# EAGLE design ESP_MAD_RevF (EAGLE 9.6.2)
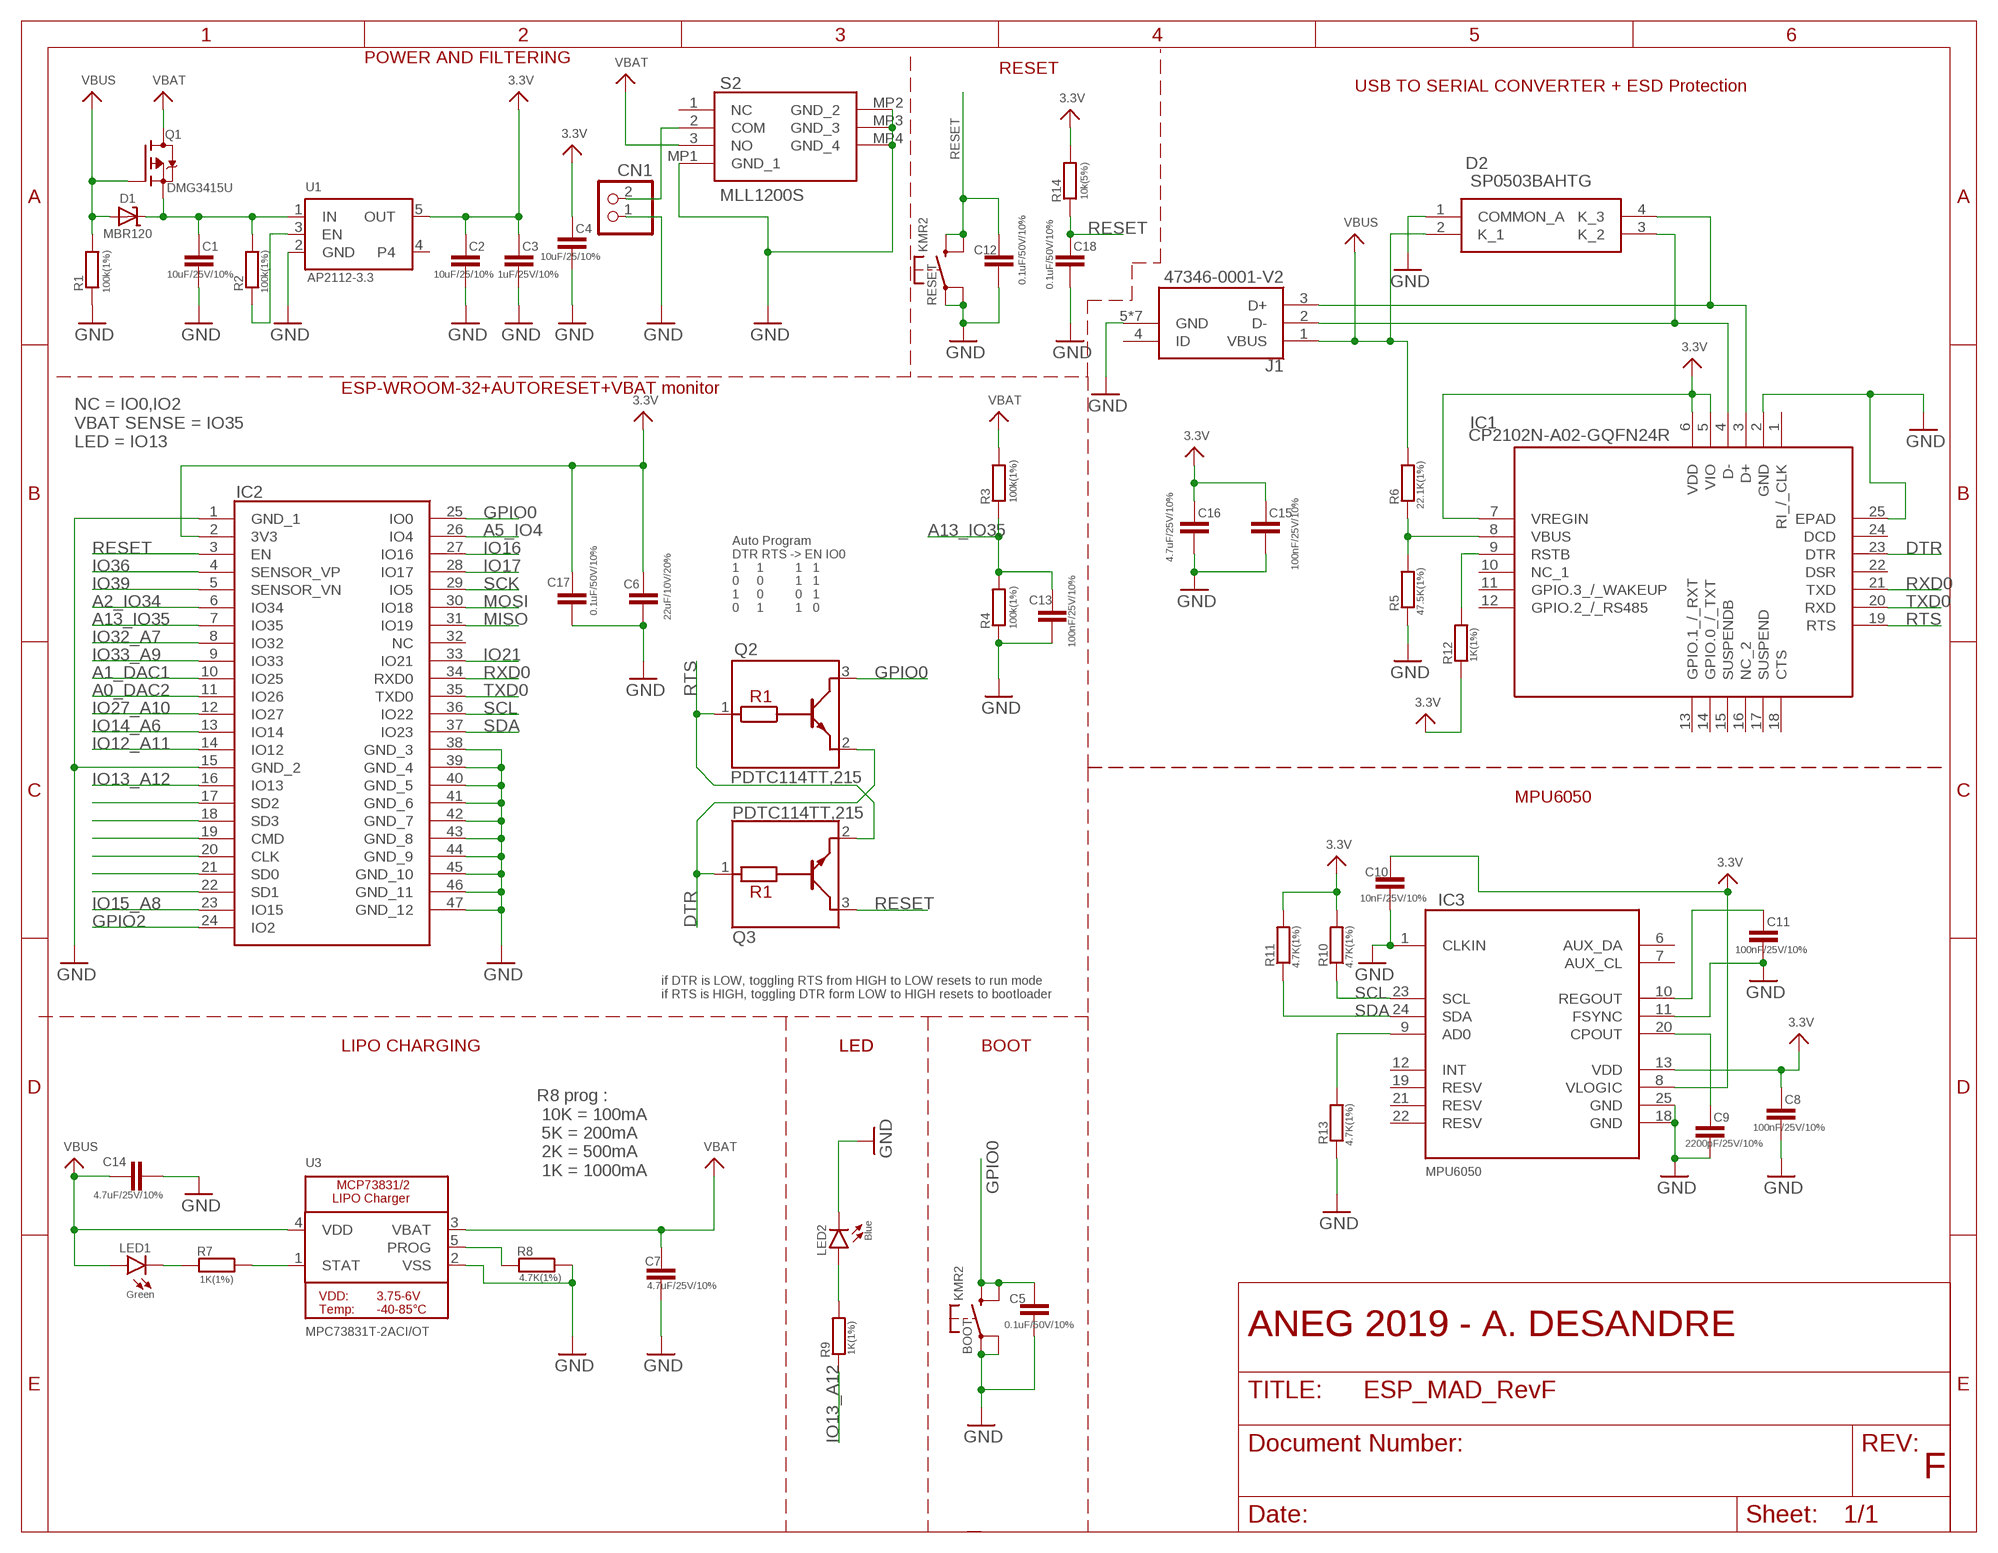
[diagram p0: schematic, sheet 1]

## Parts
BOOT  KMR2  MICROBUILDER_SWITCH_TACT_SMT4.6X2.8  [MICROBUILDER_BTN_KMR2_4.6X2.8]
C1  10uF/25V/10%  C-EUC0603  [C0603]
C2  10uF/25/10%  C-EUC0603  [C0603]
C3  1uF/25V/10%  C-EUC0603  [C0603]
C4  10uF/25/10%  C-EUC0603  [C0603]
C5  0.1uF/50V/10%  C-EUC0603  [C0603]
C6  22uF/10V/20%  C-EUC0603  [C0603]
C7  4.7uF/25V/10%  C-EUC0603  [C0603]
C8  100nF/25V/10%  C-EUC0603  [C0603]
C9  2200pF/25V/10%  C-EUC0603  [C0603]
C10  10nF/25V/10%  C-EUC0603  [C0603]
C11  100nF/25V/10%  C-EUC0603  [C0603]
C12  0.1uF/50V/10%  C-EUC0603  [C0603]
C13  100nF/25V/10%  C-EUC0603  [C0603]
C14  4.7uF/25V/10%  C-EUC0603  [C0603]
C15  100nF/25V/10%  C-EUC0603  [C0603]
C16  4.7uF/25V/10%  C-EUC0603  [C0603]
C17  0.1uF/50V/10%  C-EUC0603  [C0603]
C18  0.1uF/50V/10%  C-EUC0603  [C0603]
CN1  JST_2PIN-SMT-RA  [JST-PH-2-SMT-RA]
D1  MBR120  MICROBUILDER_DIODE-SCHOTTKYSOD-123  [MICROBUILDER_SOD-123]
D2  SP0503BAHTG  [SP0503BAHTG]
IC1  CP2102N-A02-GQFN24R  [QFN50P400X400X80-25N]
IC2  ESP32-WROOM-32D_M113DH3200PS3Q  [ESP32WROOM32DM113DH3200PS3Q0]
IC3  MPU6050  [QFN50P400X400X95-25T265X275N]
J1  47346-0001-V2  [47346-0001-V2]
LED1  Green  LEDCHIP-LED0603  [CHIP-LED0603]
LED2  Blue  LEDCHIP-LED0603  [CHIP-LED0603]
Q1  DMG3415U  MICROBUILDER_MOSFET-P  [MICROBUILDER_SOT23-R]
Q2  PDTC114TT,215  [SOT95P230X110-3N]
Q3  PDTC114TT,215  [SOT95P230X110-3N]
R1  100k(1%)  R-EU_R0603  [R0603]
R2  100k(1%)  R-EU_R0603  [R0603]
R3  100k(1%)  R-EU_R0603  [R0603]
R4  100k(1%)  R-EU_R0603  [R0603]
R5  47.5K(1%)  R-EU_R0603  [R0603]
R6  22.1K(1%)  R-EU_R0603  [R0603]
R7  1K(1%)  R-EU_R0603  [R0603]
R8  4.7K(1%)  R-EU_R0603  [R0603]
R9  1K(1%)  R-EU_R0603  [R0603]
R10  4.7K(1%)  R-EU_R0603  [R0603]
R11  4.7K(1%)  R-EU_R0603  [R0603]
R12  1K(1%)  R-EU_R0603  [R0603]
R13  4.7K(1%)  R-EU_R0603  [R0603]
R14  10k(5%)  R-EU_R0603  [R0603]
RESET  KMR2  MICROBUILDER_SWITCH_TACT_SMT4.6X2.8  [MICROBUILDER_BTN_KMR2_4.6X2.8]
S2  MLL1200S  [MLL1200S]
U1  AP2112-3.3  MICROBUILDER_VREG_SOT23-5  [MICROBUILDER_SOT23-5]
U3  MPC73831T-2ACI/OT  MICROBUILDER_MCP73831/2  [MICROBUILDER_SOT23-5]

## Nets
3.3V: C2.1 C3.1 C4.1 C6.1 C8.1 C10.1 C15.1 C16.1 C17.1 IC1.5(VIO) IC1.6(VDD) IC1.7(VREGIN) IC2.2(3V3) IC3.8(VLOGIC) IC3.13(VDD) R10.2 R11.2 R12.1 R14.2 U1.5(OUT)
A0_DAC2: IC2.11(IO26)
A1_DAC1: IC2.10(IO25)
A2_IO34: IC2.6(IO34)
A5_IO4: IC2.26(IO4)
A13_IO35: C13.1 IC2.7(IO35) R3.1 R4.2
DTR: IC1.23(DTR) Q2.2(E) Q3.1(B)
GND: BOOT.A'(P1) BOOT.A(P) C1.2 C2.2 C3.2 C4.2 C5.2 C6.2 C7.2 C8.2 C9.2 C10.2 C11.2 C12.2 C13.2 C14.2 C15.2 C16.2 C17.2 C18.2 CN1.1 D2.1(COMMON_A) IC1.2(GND) IC1.25(EPAD) IC2.1(GND_1) IC2.15(GND_2) IC2.38(GND_3) IC2.39(GND_4) IC2.40(GND_5) IC2.41(GND_6) IC2.42(GND_7) IC2.43(GND_8) IC2.44(GND_9) IC2.45(GND_10) IC2.46(GND_11) IC2.47(GND_12) IC3.1(CLKIN) IC3.11(FSYNC) IC3.18(GND) IC3.25(GND) J1.5(GND) J1.6(GND) J1.7(GND) J1.8(GND) J1.9(GND) J1.10(GND) J1.11(GND) LED2.C R1.1 R4.1 R5.1 R8.1 R13.1 RESET.A'(P1) RESET.A(P) S2.MP1(GND_1) S2.MP2(GND_2) S2.MP3(GND_3) S2.MP4(GND_4) U1.2(GND) U3.2(VSS)
GPIO0: BOOT.B'(S1) BOOT.B(S) C5.1 IC2.25(IO0) Q2.3(C)
GPIO2: IC2.24(IO2)
IO12_A11: IC2.14(IO12)
IO13_A12: IC2.16(IO13) R9.1
IO14_A6: IC2.13(IO14)
IO15_A8: IC2.23(IO15)
IO16: IC2.27(IO16)
IO17: IC2.28(IO17)
IO21: IC2.33(IO21)
IO27_A10: IC2.12(IO27)
IO32_A7: IC2.8(IO32)
IO33_A9: IC2.9(IO33)
IO36: IC2.4(SENSOR_VP)
IO39: IC2.5(SENSOR_VN)
MISO: IC2.31(IO19)
MOSI: IC2.30(IO18)
N$1: CN1.2 S2.2(COM)
N$2: R2.1 U1.3(EN)
N$3: IC2.17(SD2)
N$4: IC1.8(VBUS) R5.2 R6.1
N$5: LED1.C R7.2
N$6: R7.1 U3.1(STAT)
N$7: D2.3(K_2) IC1.4(D-) J1.2(D-)
N$8: C1.1 D1.C Q1.2(S) R2.2 U1.1(IN)
N$9: R8.2 U3.5(PROG)
N$10: C9.1 IC3.20(CPOUT)
N$11: LED2.A R9.2
N$12: D2.4(K_3) IC1.3(D+) J1.3(D+)
N$13: C11.1 IC3.10(REGOUT)
N$14: IC1.9(RSTB) R12.2
N$15: IC2.18(SD3)
N$16: IC2.19(CMD)
N$17: IC2.20(CLK)
N$18: IC2.21(SD0)
N$19: IC2.22(SD1)
N$20: IC3.9(AD0) R13.2
RESET: C12.1 C18.1 IC2.3(EN) Q3.3(C) R14.1 RESET.B'(S1) RESET.B(S)
RTS: IC1.19(RTS) Q2.1(B) Q3.2(E)
RXD0: IC1.21(TXD) IC2.34(RXD0)
SCK: IC2.29(IO5)
SCL: IC2.36(IO22) IC3.23(SCL) R10.1
SDA: IC2.37(IO23) IC3.24(SDA) R11.1
TXD0: IC1.20(RXD) IC2.35(TXD0)
VBAT: C7.1 Q1.3(D) R3.2 S2.3(NO) U3.3(VBAT)
VBUS: C14.1 D1.A D2.2(K_1) J1.1(VBUS) LED1.A Q1.1(G) R1.2 R6.2 U3.4(VDD)
Unconnected: IC1.1(RI_/_CLK) IC1.10(NC_1) IC1.11(GPIO.3_/_WAKEUP) IC1.12(GPIO.2_/_RS485) IC1.13(GPIO.1_/_RXT) IC1.14(GPIO.0_/_TXT) IC1.15(SUSPENDB) IC1.16(NC_2) IC1.17(SUSPEND) IC1.18(CTS) IC1.22(DSR) IC1.24(DCD) IC2.32(NC) IC3.2(NC) IC3.3(NC) IC3.4(NC) IC3.5(NC) IC3.6(AUX_DA) IC3.7(AUX_CL) IC3.12(INT) IC3.14(NC) IC3.15(NC) IC3.16(NC) IC3.17(NC) IC3.19(RESV) IC3.21(RESV) IC3.22(RESV) J1.4(ID) S2.1(NC) U1.4

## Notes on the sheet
- POWER AND FILTERING
- RESET
- USB TO SERIAL CONVERTER + ESD Protection
- ESP-WROOM-32+AUTORESET+VBAT monitor
- NC = IO0,IO2
  VBAT SENSE = IO35
  LED = IO13
- Auto Program
  DTR RTS -> EN IO0
  1     1         1   1
  0     0         1   1
  1     0         0   1
  0     1         1   0
- MPU6050
- if DTR is LOW, toggling RTS from HIGH to LOW resets to run mode
  if RTS is HIGH, toggling DTR form LOW to HIGH resets to bootloader
- LIPO CHARGING | LED | LED | BOOT
- R8 prog :
   10K = 100mA
   5K = 200mA
   2K = 500mA
   1K = 1000mA
- ANEG 2019 | ANEG 2019 - A. DESANDRE
- F

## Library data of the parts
BOOT RESET = Adafruit HUZZAH32 ESP32 Feather:MICROBUILDER_SWITCH_TACT_SMT: SMT Tact Switches 6x6mm - Digikey: P12940SCT-ND KMR2 (4.6x2.8mm) - Digikey: 401-1426-1-ND EVQ-PQHB55 - Light Touch, 160GF (4.5x4.5mm) - Digikey: P8090SCT-ND KMT0 - KMT021 NGJ LHS (etc.) IP68/Waterproof - Digikey: CKN10289CT-ND; MANUFACTURER: C&K; MANUFACTURER_PART_NUMBER: KMR211NGLFS; MOUSER_PART_NUMBER: 611-KMR211NG-LFS; UNIT_PRICE: 0,49
C1 C2 C4 = rcl:C-EU: CAPACITOR, European symbol; MANUFACTURER: MURATA; MANUFACTURER_PART_NUMBER: GRM188R61E106KA73D; MOUSER_PART_NUMBER: 81-GRM188R61E106KA3D; PACKAGE: 0603; SPICEPREFIX: C; UNIT_PRICE: 0,324
C3 = rcl:C-EU: CAPACITOR, European symbol; MANUFACTURER: MURATA; MANUFACTURER_PART_NUMBER: GCJ188R71E105KA01D; MOUSER_PART_NUMBER: 81-GCJ188R71E105KA1D; PACKAGE: 0603; SPICEPREFIX: C; UNIT_PRICE: 0,252
C5 C12 C17 C18 = rcl:C-EU: CAPACITOR, European symbol; MANUFACTURER: MURATA; MANUFACTURER_PART_NUMBER: GCJ188R71H104KA12D; MOUSER_PART_NUMBER: 81-GCJ188R71H104KA2D; PACKAGE: 0603; SPICEPREFIX: C; UNIT_PRICE: 0,2
C6 = rcl:C-EU: CAPACITOR, European symbol; MANUFACTURER: MURATA; MANUFACTURER_PART_NUMBER: GRT188R61A226ME13D; MOUSER_PART_NUMBER: 81-GRT188R61A226ME13; PACKAGE: 0603; SPICEPREFIX: C; UNIT_PRICE: 0,46
C7 C14 C16 = rcl:C-EU: CAPACITOR, European symbol; MANUFACTURER: MURATA; MANUFACTURER_PART_NUMBER: GRT188C81E475KE13D; MOUSER_PART_NUMBER: 81-GRT188C81E475KE3D; PACKAGE: 0603; SPICEPREFIX: C; UNIT_PRICE: 0,43
C8 C11 C13 C15 = rcl:C-EU: CAPACITOR, European symbol; MANUFACTURER: MURATA; MANUFACTURER_PART_NUMBER: GCJ188R71E104KA12D; MOUSER_PART_NUMBER: 81-GCJ188R71E104KA2D; PACKAGE: 0603; SPICEPREFIX: C; UNIT_PRICE: 0,18
C9 = rcl:C-EU: CAPACITOR, European symbol; MANUFACTURER: MURATA; MANUFACTURER_PART_NUMBER: GCJ188R71E222KA01D; MOUSER_PART_NUMBER: 81-GCJ188R71E222KA1D; PACKAGE: 0603; SPICEPREFIX: C; UNIT_PRICE: 0,153
C10 = rcl:C-EU: CAPACITOR, European symbol; MANUFACTURER: MURATA; MANUFACTURER_PART_NUMBER: GCJ188R71E103KA01D; MOUSER_PART_NUMBER: 81-GCJ188R71E103KA1D; PACKAGE: 0603; SPICEPREFIX: C; UNIT_PRICE: 0,144
CN1 = adafruit:JST_2PIN: JST 2-Pin Connectors of various flavors; MANUFACTURER: ADAFRUIT; MANUFACTURER_PART_NUMBER: 1769; MOUSER_PART_NUMBER: 485-1769; UNIT_PRICE: 0,68
D1 = Adafruit HUZZAH32 ESP32 Feather:MICROBUILDER_DIODE-SCHOTTKY; FARNELL_PART_NUMBER: 2533227; MANUFACTURER_PART_NUMBER: MBR120VLSFT3G; MOUSER_PART_NUMBER: 863-MBR120VLSFT3G; PACKAGE: SOD-123FL; UNIT_PRICE: 0,351
D2 = SamacSys_Parts:SP0503BAHTG: ESD Suppressors / TVS Diodes TVS AVAL DIODE SMT Source: Datasheet; DESCRIPTION: ESD Suppressors / TVS Diodes TVS AVAL DIODE SMT; HEIGHT: 1.22mm; MANUFACTURER_NAME: LITTELFUSE; MANUFACTURER_PART_NUMBER: SP0503BAHTG; MOUSER_PART_NUMBER: 576-SP0503BAHTG; MOUSER_PRICE-STOCK: https://www.mouser.co.uk/ProductDetail/Littelfuse/SP0503BAHTG?qs=uD%2FdkN7XIa0NTYXwHdELYA%3D%3D; UNIT_PRICE: 0,68
IC1 = SamacSys_Parts:CP2102N-A02-GQFN24R: USB Interface IC USB to UART bridge - QFN24 Source: Datasheet; DESCRIPTION: USB Interface IC USB to UART bridge - QFN24; HEIGHT: 0.8mm; MANUFACTURER_NAME: Silicon Labs; MANUFACTURER_PART_NUMBER: CP2102N-A02-GQFN24R; MOUSER_PART_NUMBER: 634-CP2102NA02QFN24R; MOUSER_PRICE-STOCK: https://www.mouser.co.uk/ProductDetail/Silicon-Labs/CP2102N-A02-GQFN24R?qs=u16ybLDytRaIVBf0X4zL0g%3D%3D; UNIT_PRICE: 1,14
IC2 = SamacSys_Parts:ESP32-WROOM-32D_M113DH3200PS3Q: WiFi Modules (802.11) ESP32-WROOM-32D Automotive PCB ANT Source: Datasheet; DESCRIPTION: WiFi Modules (802.11) ESP32-WROOM-32D Automotive PCB ANT; HEIGHT: 3.2mm; MANUFACTURER_NAME: Espressif Systems; MANUFACTURER_PART_NUMBER: ESP32-WROOM-32D(M113DH3200PS3Q0); MOUSER_PART_NUMBER: 356-ESPWROOM3200PS3; MOUSER_PRICE-STOCK: https://www.mouser.co.uk/ProductDetail/Espressif-Systems/ESP32-WROOM-32DM113DH3200PS3Q0?qs=wnTfsH77Xs7iNQbBNob0RQ%3D%3D; UNIT_PRICE: 3,30
IC3 = invensense:MPU6050: The triple-axis MEMS gyroscope; FARNELL_PART_NUMBER: 1864742; MANUFACTURER_PART_NUMBER: MPU-6050; MOUSER_PART_NUMBER: 410-MPU-6050; UNIT_PRICE: 6,55
J1 = SamacSys_Parts:47346-0001-V2; MANUFACTURER_PART_NUMBER: 47346-1001; MOUSER_PART_NUMBER: 538-47346-1001; PACKAGE: Molex; SPICEPREFIX: M; UNNIT_PRICE: 0,81
LED1 = led:LED: LED; MANUFACTURER: BROADCOM/AVAGO; MANUFACTURER_PART_NUMBER: HSMQ-C191-T0000; MOUSER_PART_NUMBER: 630-HSMQ-C191-T0000; PACKAGE: 0603; UNIT_PRICE: 0,89
LED2 = led:LED: LED; MANUFACTURER: BROADCOM/Avago; MANUFACTURER_PART_NUMBER: HSMR-C191-S0000; MOUSER_PART_NUMBER: 630-HSMR-C191-S0000; PACKAGE: 0603; UNIT_PRICE: 0,72
Q1 = Adafruit HUZZAH32 ESP32 Feather:MICROBUILDER_MOSFET-P: P-Channel Mosfet LEGEND VDS: Voltage Drain-Source ID: Drain Current RDS(ON): Drain-Source On-State Resistance VGS(TH): Gate-Source Threshold Voltage CISS: Drain-Source Input Capacitance SOT-23 Name VDS ID RDS(ON) VGS(TH) CISS Order Number IRLML5103 30V 760mA 600 mOhm -- 75pF @ 25V Digikey: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; FARNELL_PART_NUMBER: 1843688RL; MANUFACTURER_PART_NUMBER: DMG3415U-7; MOUSER_PART_NUMBER: 621-DMG3415U-7; PACKAGE: SOT23; UNIT_PRICE: 0,39
Q2 Q3 = SamacSys_Parts:PDTC114TT,215: Bipolar Transistors - Pre-Biased TRANS RET TAPE-7 Source: Datasheet; DESCRIPTION: Bipolar Transistors - Pre-Biased TRANS RET TAPE-7; HEIGHT: 1.1mm; MANUFACTURER_NAME: Nexperia; MANUFACTURER_PART_NUMBER: PDTC114TT,215; MOUSER_PART_NUMBER: 771-PDTC114TT215; MOUSER_PRICE-STOCK: https://www.mouser.com/Search/Refine.aspx?Keyword=771-PDTC114TT215; UNIT_PRICE: 0,141
R1-R4 = rcl:R-EU_: RESISTOR, European symbol; MANUFACTURER_PART_NUMBER: ASC0603-100KFT5; MOUSER_PART_NUMBER: 756-ASC0603-100KFT5; PACKAGE: 0603; SPICEPREFIX: R; UNIT_PRICE: 0,272
R5 = rcl:R-EU_: RESISTOR, European symbol; MANUFACTURER_PART_NUMBER: RT0603FRE0747K5L; MOUSER_PART_NUMBER: 603-RT0603FRE0747K5L; PACKAGE: 0603; SPICEPREFIX: R; UNIT_PRICE: 0,16
R6 = rcl:R-EU_: RESISTOR, European symbol; MANUFACTURER_PART_NUMBER: RT0603FRE0722K1L; MOUSER_PART_NUMBER: 603-RT0603FRE0722K1L; PACKAGE: 0603; SPICEPREFIX: R; UNIT_PRICE: 0,16
R7 R9 R12 = rcl:R-EU_: RESISTOR, European symbol; MANUFACTURER_PART_NUMBER: RN73R1JTTD1001F50; MOUSER_PART_NUMBER: 660-RN73R1JTD1001F50; PACKAGE: 0603; SPICEPREFIX: R; UNIT_PRICE: 0,43
R8 R10 R11 R13 = rcl:R-EU_: RESISTOR, European symbol; MANUFACTURER_PART_NUMBER: RN73H1JTTD4701F100; MOUSER_PART_NUMBER: 660-RN73H1JT4701F100; PACKAGE: 0603; SPICEPREFIX: R; UNIT_PRICE: 0,221
R14 = rcl:R-EU_: RESISTOR, European symbol; MANUFACTURER_PART_NUMBER: RN73R1JTTD1002F50; MOUSER_PART_NUMBER: 660-RN73R1JTD1002F50; PACKAGE: 0603; SPICEPREFIX: R; UNIT_PRICE: 0,433
S2 = SamacSys_Parts:MLL1200S: TE CONNECTIVITY / ALCOSWITCH - MLL1200S - SLIDE SWITCH, SPDT, 0.3A, 4VDC, SMD Source: Datasheet; DESCRIPTION: TE CONNECTIVITY / ALCOSWITCH - MLL1200S - SLIDE SWITCH, SPDT, 0.3A, 4VDC, SMD; FARNELL_PART_NUMBER: 2749889; HEIGHT: 1.75mm; MANUFACTURER_NAME: TE Connectivity; MANUFACTURER_PART_NUMBER: MLL1200S; MOUSER_PART_NUMBER: 506-MLL1200S; MOUSER_PRICE-STOCK: https://www.mouser.com/Search/Refine.aspx?Keyword=506-MLL1200S; UNIT_PRICE: 2,13
U1 = Adafruit HUZZAH32 ESP32 Feather:MICROBUILDER_VREG_SOT23-5: SOT23-5 Fixed Voltage Regulators Part Current Out V Out V In V Dropout θJA (°C/W) TJ (°C) Digikey Part No. ADP121 150mA 3.3V 3.4-5.5V 0.09V @ 150mA -- -- ADP121-AUJZ33R7CT-ND ADP121 150mA 3.0V 3.1-5.5V 0.09V @ 150mA -- -- ADP121-AUJZ30R7CT-ND ADP122 300mA 3.3V 3.4-5.5V 0.085V @ 300mA -- --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; FARNELL: AP2112K-3.3TRG1DICT-ND; MANUFACTURER_PART_NUMBER: AP2112K-3.3TRG1; MOUSER_PART_NUMBER: 621-AP2112K-3.3TRG1; PACKAGE: SOT25; UNIT_PRICE: 0,42
U3 = Adafruit HUZZAH32 ESP32 Feather:MICROBUILDER_MCP73831/2: MCP73831/2 LIPO Charger VDD: 3.75 - 6V Temp -40 - 85°C Programmable Charge Rate: 15-500mA NOTE: STAT is a tri-state logic output on the MCP73831 and an open-drain output on the MCP73832. SOT23-5 with 4.2V output and tri-state logic on STAT = MCP73831T-2ACI/OT; FARNELL_PART_NUMBER: 1332158; MANUFACTURER_PART_NUMBER: MCP73831T-2ACI/OT; MOUSER_PART_NUMBER: 579-MCP73831T-2ACIOT; PACKAGE: SOT25; UNIT_PRICE: 0,49

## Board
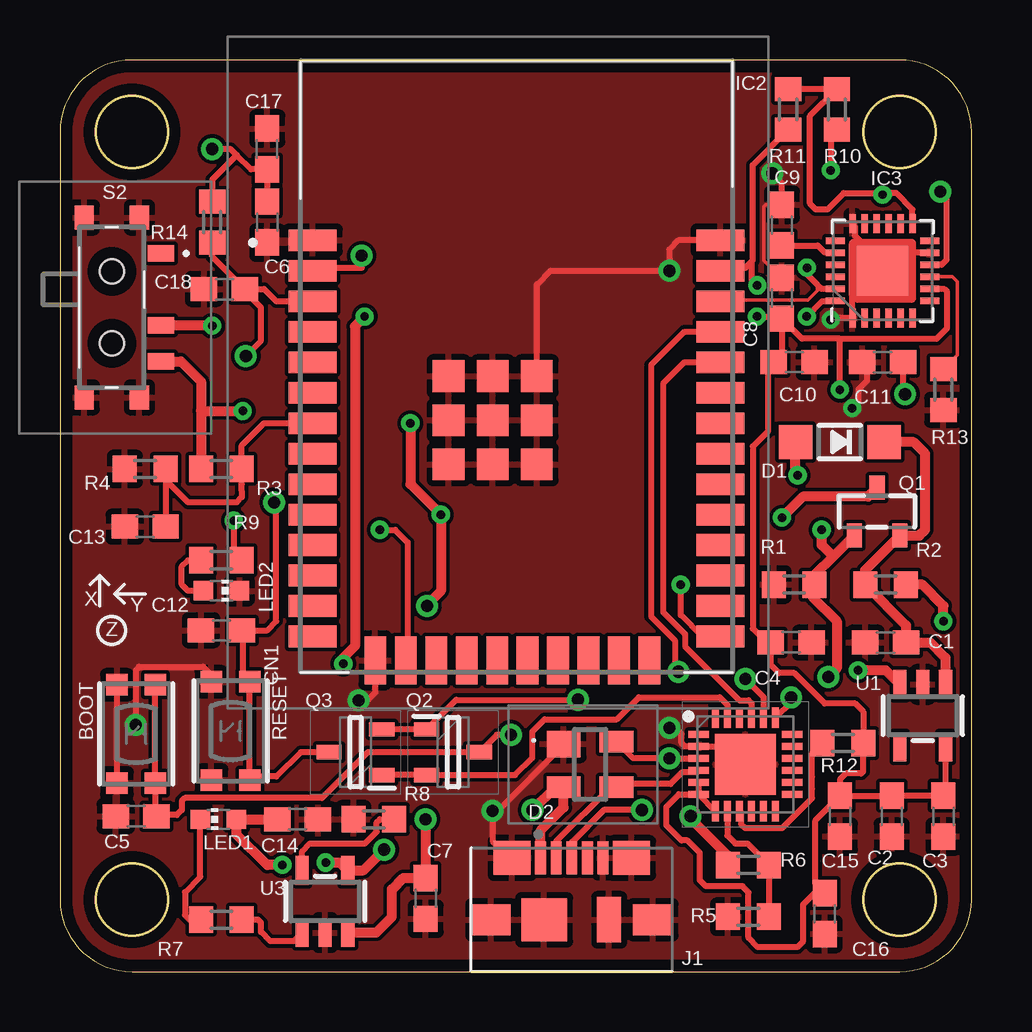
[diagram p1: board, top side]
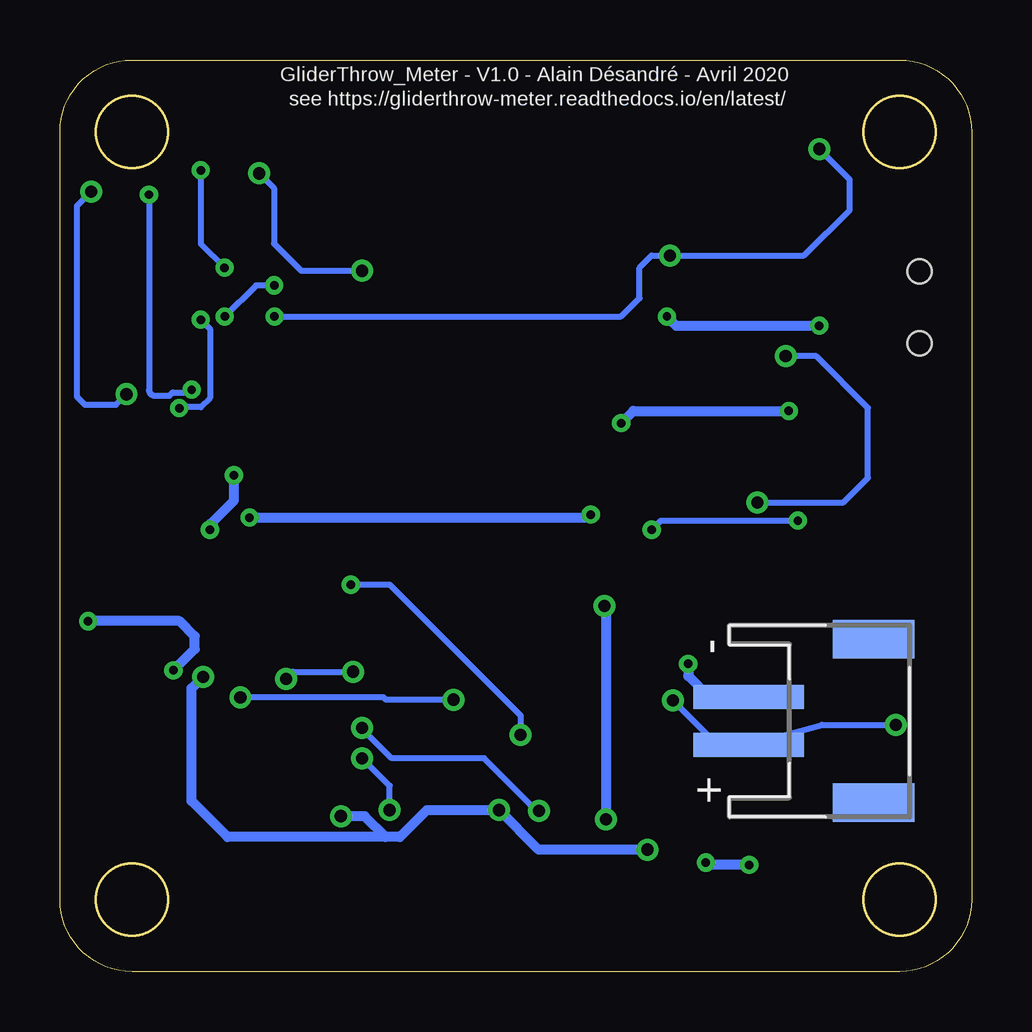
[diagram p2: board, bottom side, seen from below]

Size 38 x 38 mm. Coordinates in mm from the lower left corner, seen from the top.
Outline: 3,0 35,0 arc90 38,3 38,35 arc90 35,38 3,38 arc90 0,35 0,3 arc90 3,0
Outline: circle at 3,3 radius 1.5
Outline: circle at 35,35 radius 1.5
Outline: circle at 35,3 radius 1.5
Outline: circle at 3,35 radius 1.5
Copper layers (1*16): Top 0.035mm / dielectric 1.5mm / Bottom 0.035mm
Design rules "default *": minimum track width 6mil, minimum drill 0.35mm, track to track 6mil, track to pad 6mil, pad to pad 6mil, via to via 6mil, smd to smd 6mil, copper to edge 20mil, drill to drill 6mil, minimum pad ring 10mil, minimum via ring 8mil, stop-mask expansion 4mil, vias tented up to drill 0mil, thermal gap 10mil

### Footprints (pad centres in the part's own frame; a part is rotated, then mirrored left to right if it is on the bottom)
MICROBUILDER_BTN_KMR2_4.6X2.8 = smd 0.9 x 0.9: A 2.05,0.8; A' -2.05,0.8; B 2.05,-0.8; B' -2.05,-0.8
C0603 = smd 1.1 x 1: 1 -0.85,0; 2 0.85,0
JST-PH-2-SMT-RA = smd 1 x 4.6: 1 1,-3.7; 2 -1,-3.7 | smd 1.6 x 3.4: NC1 -3.4,1.5; NC2 3.4,1.5
MICROBUILDER_SOD-123 = smd 1.4 x 1.4: A 1.85,0; C -1.85,0
SP0503BAHTG = smd 1.1 x 1.4: 1 -0.85,-1.1 | smd 0.9 x 1.4: 2 0.95,-1.1; 3 0.95,1.1; 4 -0.95,1.1
QFN50P400X400X80-25N = smd 0.85 x 0.3: 1 -1.95,1.25; 2 -1.95,0.75; 3 -1.95,0.25; 4 -1.95,-0.25; 5 -1.95,-0.75; 6 -1.95,-1.25; 13 1.95,-1.25; 14 1.95,-0.75; 15 1.95,-0.25; 16 1.95,0.25; 17 1.95,0.75; 18 1.95,1.25 | smd 0.3 x 0.85: 7 -1.25,-1.95; 8 -0.75,-1.95; 9 -0.25,-1.95; 10 0.25,-1.95; 11 0.75,-1.95; 12 1.25,-1.95; 19 1.25,1.95; 20 0.75,1.95; 21 0.25,1.95; 22 -0.25,1.95; 23 -0.75,1.95; 24 -1.25,1.95 | smd 2.55 x 2.55: 25 0,0
ESP32WROOM32DM113DH3200PS3Q0 = smd 2 x 0.9: 1 0,0; 2 0,-1.27; 3 0,-2.54; 4 0,-3.81; 5 0,-5.08; 6 0,-6.35; 7 0,-7.62; 8 0,-8.89; 9 0,-10.16; 10 0,-11.43; 11 0,-12.7; 12 0,-13.97; 13 0,-15.24; 14 0,-16.51; 25 17,-16.51; 26 17,-15.24; 27 17,-13.97; 28 17,-12.7; 29 17,-11.43; 30 17,-10.16; 31 17,-8.89; 32 17,-7.62; 33 17,-6.35; 34 17,-5.08; 35 17,-3.81; 36 17,-2.54; 37 17,-1.27; 38 17,0 | smd 0.9 x 2: 15 2.6,-17.51; 16 3.87,-17.51; 17 5.14,-17.51; 18 6.41,-17.51; 19 7.68,-17.51; 20 8.95,-17.51; 21 10.22,-17.51; 22 11.49,-17.51; 23 12.76,-17.51; 24 14.03,-17.51 | smd 1.33 x 1.33: 39 5.665,-5.665; 40 7.5,-5.665; 41 9.335,-5.665; 42 5.665,-7.5; 43 7.5,-7.5; 44 9.335,-7.5; 45 5.665,-9.335; 46 7.5,-9.335; 47 9.335,-9.335
QFN50P400X400X95-25T265X275N = smd 0.26 x 0.79: 1 -1.25,-1.97; 2 -0.75,-1.97; 3 -0.25,-1.97; 4 0.25,-1.97; 5 0.75,-1.97; 6 1.25,-1.97; 13 1.25,1.97; 14 0.75,1.97; 15 0.25,1.97; 16 -0.25,1.97; 17 -0.75,1.97; 18 -1.25,1.97 | smd 0.79 x 0.26: 7 1.97,-1.25; 8 1.97,-0.75; 9 1.97,-0.25; 10 1.97,0.25; 11 1.97,0.75; 12 1.97,1.25; 19 -1.97,1.25; 20 -1.97,0.75; 21 -1.97,0.25; 22 -1.97,-0.25; 23 -1.97,-0.75; 24 -1.97,-1.25 | smd 2.15 x 2.05: 25 0,0
47346-0001-V2 = smd 0.45 x 1.38: 1 -1.3,2.575; 2 -0.65,2.575; 3 0,2.575; 4 0.65,2.575; 5 1.3,2.575 | smd 1.55 x 1.425: 6 2.487,2.575; 11 -2.487,2.575 | smd 1.65 x 1.3: 7 3.375,0; 10 -3.376,0 | smd 1 x 1.9: 8 1.55,0 | smd 1.9 x 1.8: 9 -1.15,0
CHIP-LED0603 = smd 0.8 x 0.8: A 0,-0.75; C 0,0.75
MICROBUILDER_SOT23-R = smd 0.635 x 1.016: 1 -0.95,-1; 2 0.95,-1; 3 0,1
SOT95P230X110-3N = smd 1.05 x 0.6: 1 -1.1,0.95; 2 -1.1,-0.95; 3 1.1,0
R0603 = smd 1 x 1.1: 1 -0.85,0; 2 0.85,0
MLL1200S = smd 0.7 x 1.1: 1 -2.25,2.05; 2 0.75,2.05; 3 2.25,2.05 | smd 1 x 0.8: MP1 -3.75,1.15; MP2 3.75,1.15; MP3 3.75,-1.15; MP4 -3.75,-1.15 | hole 1: -1.5,0; 1.5,0
MICROBUILDER_SOT23-5 = smd 0.55 x 1.2: 1 -0.95,-1.3; 2 0,-1.3; 3 0.95,-1.3; 4 0.95,1.3; 5 -0.95,1.3

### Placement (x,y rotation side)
BOOT  3.17,9.91 90 top
C1  34.42,13.72 180 top
C2  34.67,6.48 270 top
C3  36.83,6.48 270 top
C4  30.48,13.72 0 top
C5  3.17,6.48 180 top
C6  8.64,31.24 270 top
C7  15.24,3.05 270 top
C8  30.1,28.07 90 top
C9  30.1,31.11 90 top
C10  30.61,25.4 0 top
C11  34.29,25.4 180 top
C12  6.73,14.22 180 top
C13  3.56,18.54 180 top
C14  9.91,6.35 0 top
C15  32.51,6.48 270 top
C16  31.88,2.41 270 top
C17  8.64,34.29 90 top
C18  6.86,28.45 180 top
CN1  5.58,10.45 270 bottom
D1  32.51,22.07 180 top
D2  22.1,8.64 270 top
IC1  28.57,8.64 0 top
IC2  10.54,30.48 0 top
IC3  34.29,29.21 0 top
J1  21.34,2.16 0 top
LED1  6.6,6.35 90 top
LED2  6.73,15.88 270 top
Q1  34.06,19.18 0 top
Q2  16.38,9.14 0 top
Q3  12.32,9.14 180 top
R1  30.61,16.13 0 top
R2  34.42,16.13 180 top
R3  6.73,20.95 180 top
R4  3.56,20.95 0 top
R5  28.7,2.29 0 top
R6  28.7,4.45 180 top
R7  6.73,2.16 180 top
R8  13.08,6.35 0 top
R9  6.73,17.14 180 top
R10  32.38,35.94 90 top
R11  30.35,35.94 90 top
R12  32.64,9.53 180 top
R13  36.83,24.26 90 top
R14  6.35,31.24 90 top
RESET  7.11,10.03 90 top
S2  2.16,27.69 270 top
U1  35.97,10.67 180 top
U3  11.05,2.92 0 top

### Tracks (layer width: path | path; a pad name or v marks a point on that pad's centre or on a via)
3.3V  (via drill 0.35, 0.51)
  Top 0.254: R11.2 R10.2 31.27,35.68 31.27,32.01 31.5,31.78 32,31.78 32.67,32.45 34.35,32.45 | U1.5 36.92,7.41 C3.1 C2.1 C15.1 | v29.06,27.3 30.01,27.3 C8.1 | C8.1 30.1,25.74 C10.1 29.5,25.15 29.5,22.51 28.88,21.89 28.88,14.3 29.46,13.72 C4.1 29.63,12.79 29.97,12.45 30.61,12.45 31.88,11.18 33.15,11.18 33.49,10.83 R12.1 33.49,8.34 33.4,8.26 32.77,8.26 32.51,8 C15.1 | IC3.8 36.27,28.45 36.88,28.45 36.98,28.34 36.98,26.82 36.55,26.39 36.55,26.38 32.51,26.38 | 34.35,32.45 v34.29,32.38 | v32.51,24.26 32.51,26.38 | v12.57,29.84 12.57,29.34 10.67,29.34 IC2.2 | C6.1 C17.1 7.96,33.44 7.37,34.04 | C15.1 31.5,6.31 31.5,3.64 C16.1 31.46,3.26 30.99,2.79 30.99,1.27 30.73,1.02 29.08,1.02 28.7,1.4 28.7,3.3 28.45,3.56 26.92,3.56 26.67,3.81 26.67,4.95 26.16,5.46 25.91,5.46 25.27,6.1 25.27,6.86 25.8,7.39 IC1.6 | IC1.6 IC1.5 | IC1.6 IC1.7 | v6.35,34.29 7.11,34.29 7.37,34.04 | IC3.13 35.54,31.77 34.86,32.45 34.35,32.45 | 7.37,34.04 6.35,33.02 R14.2 | C8.1 30.93,26.38 32.51,26.38
  Bottom 0.254: v34.29,32.38 34.29,24.26 arc-90 34.04,24 33.44,24 33.3,24.14 32.62,24.14 v32.51,24.26 | v6.35,34.29 5.08,33.02 5.08,31.75 6.99,29.84 v12.57,29.84 13.34,29.84 13.84,29.34 13.84,28.07 14.61,27.3 v29.06,27.3
A13_IO35
  Top 0.254: R4.2 4.41,20.83 4.41,20.49 | 4.41,20.49 C13.1 | IC2.7 8.51,22.86 7.58,21.93 R3.1 7.58,20.32 7.58,20.03 7.58,19.77 7.37,19.56 5.33,19.56 4.41,20.49
DTR
  Top 0.254: Q3.1 Q2.2 18.98,8.19 19.69,8.9 19.69,10 20.2,10.52 23.22,10.52 24.13,11.43 27.51,11.43 27.83,11.11 IC1.23
GND  (via drill 0.35, 0.51)
  Top 0.152: C9.2 29.43,31.96 29.34,31.88 29.34,29.63 29.52,29.44 C8.2
  Top 0.254: v32.13,27.17 32.2,27.24 IC3.1 33.04,28.26 34.29,29.51 | v33.03,23.49 33.28,23.74 33.28,24.27 33.66,24.64 33.66,25.18 C11.2 | IC1.25 28.28,8.64 27.53,9.39 27,9.39 IC1.2 26.05,9.39 25.91,9.53 25.91,9.91 25.65,10.16 v25.4,10.16 | J1.11 18.73,4.73 18.03,5.43 v18.03,6.7 18.26,6.7 21,9.44 D2.1 | C9.2 30.1,32.87 v29.7,33.27 | IC2.38 25.78,30.48 25.4,30.1 v25.4,29.21 20.45,29.21 19.88,28.64 IC2.41 | BOOT.A' BOOT.A | RESET.A 6.31,12.36 5.97,12.7 3.3,12.7 3.16,12.56 v3.16,10.29 | IC3.18 33.13,31.09 33.13,30.67 34.29,29.51 | 34.29,29.51 IC3.25 35.04,29.96 IC3.11 | IC2.15 13.14,11.62 12.83,11.3 v12.45,11.3
  Bottom 0.254: v32.13,27.17 31.75,26.79 31.75,23.91 32.13,23.52 32.99,23.52 v33.03,23.49 | v18.03,6.7 18.13,6.7 20.32,8.89 24.18,8.89 25.4,10.11 v25.4,10.16 | v29.7,33.27 29.08,32.66 29.08,30.35 27.94,29.21 v25.4,29.21 | v3.16,10.29 6.22,10.29 CN1.1 10.59,9.45 v12.45,11.3
  pour Top: 1.78,0 36.2,0 37.97,1.78 37.97,36.2 36.2,37.97 2.16,37.97 0,35.81 0,2.54 0.13,2.41 0.13,1.65
GPIO0  (via drill 0.35, 0.51)
  Top 0.254: v18.8,9.87 18.21,9.87 Q2.3 12.83,9.14 10.92,7.24 5.21,7.24 5.08,7.11 5.08,6.73 4.87,6.52 3.98,6.52 | v25.88,16.13 25.88,14.86 26.76,13.97 IC2.25 | 3.98,6.52 3.98,6.53 BOOT.B' BOOT.B | 3.98,6.52 C5.1
  Bottom 0.254: v25.88,16.13 v25.87,16.13 24.26,16.13 18.8,10.67 v18.8,9.87
IO13_A12  (via drill 0.35)
  Top 0.254: v13.34,18.41 13.97,18.41 14.49,17.89 14.49,13.05 IC2.16 | R9.1 7.24,17.49 v7.24,18.8
  Bottom 0.254: v13.34,18.41 12.95,18.8 v7.24,18.8
N$1  (via drill 0.35)
  Top 0.254: v6.35,26.92 6.34,26.94
  Top 0.406: 6.34,26.94 S2.2 | v12.7,27.3 12.3,26.9 12.3,13.57 11.81,13.08 v11.81,12.83
  Bottom 0.406: v12.7,27.3 12.32,26.92 v6.35,26.92 | v11.81,12.83 11.81,12.32 10.94,11.45 CN1.2
N$2  (via drill 0.35)
  Top 0.406: U1.3 34.42,12.56 v33.27,12.56 | v36.83,14.61 36.83,15.24 35.94,16.13 R2.1
  Bottom 0.406: v33.27,12.56 32.38,13.45 32.38,13.97 33.02,14.61 v36.83,14.61
N$4
  Top 0.254: IC1.8 27.81,6.67 27.81,5.68 28.16,5.33 28.66,5.33 R6.1 R5.2
N$5
  Top 0.254: R7.2 5.75,2.03 5.53,2.03 5.21,2.35 5.21,3.31 5.85,3.95 LED1.C
N$6
  Top 0.254: U3.1 9.75,1.27 8.76,1.27 8.38,1.65 8.38,2.03 8.26,2.16 R7.1
N$7
  Top 0.254: J1.2 20.69,5.43 22.94,7.69 D2.3 23.32,7.81 25.45,7.81 25.96,8.31 26.55,8.31 IC1.4
N$8
  Top 0.406: U1.1 36.92,13.08 36.28,13.72 C1.1 35.27,14.43 R2.2 33.57,16.73 Q1.2 35.83,18.18 36.07,18.41 36.07,21.59 35.59,22.07 D1.C
N$9
  Top 0.254: U3.5 10.1,5.02 10.41,5.33 12.71,5.33 13.21,5.83 13.21,6.22 13.34,6.35 R8.2
N$10
  Top 0.254: C9.1 31.58,30.27 31.88,29.97 32.31,29.97 IC3.20
N$11
  Top 0.254: LED2.A 5.33,15.88 5.08,16.13 5.08,16.89 5.33,17.14 R9.2
N$12  (via drill 0.51)
  Top 0.254: D2.4 23.89,8.89 v25.4,8.89 IC1.3 | J1.3 21.34,5.39 22.67,6.73 v24.26,6.73
  Bottom 0.254: v24.26,6.73 24.26,7.75 v25.4,8.89
N$13  (via drill 0.51)
  Top 0.254: IC3.10 36.76,29.46 36.96,29.66 36.96,32.26 v36.7,32.51 | C11.1 35.14,24.16 v35.23,24.07
  Bottom 0.254: v35.23,24.07 35.67,23.62 36.96,23.62 37.29,23.95 37.29,31.93 v36.7,32.51
N$14
  Top 0.254: IC1.9 28.4,6.62 28.4,6.14 28.56,5.98 30.11,5.98 31.35,7.22 31.35,7.62 31.35,8.12 31.35,9.09 R12.2
N$20
  Top 0.152: IC3.9 37.21,28.96 37.42,28.75 37.42,25.69 R13.2
RESET  (via drill 0.51)
  Top 0.254: RESET.B' 7.91,8.13 | 7.91,8.13 RESET.B 7.62,12.37 7.62,14.19 C12.1 8.64,14.22 9.02,14.61 9.02,19.47 v8.93,19.56 | Q3.3 10.03,9.14 9.02,8.13 7.91,8.13 | v7.75,25.65 8.38,26.29 8.38,27.69 7.71,28.36 C18.1 | C18.1 8.51,28.45 9.02,27.94 IC2.3 | C18.1 6.35,29.81 R14.1
  Bottom 0.254: v8.93,19.56 5.33,19.56 4.32,20.57 4.32,23.5 6.48,25.65 v7.75,25.65
RTS  (via drill 0.51)
  Top 0.254: Q3.2 Q2.1 16.52,11.33 v21.59,11.33 | v30.48,11.43 30.48,11.24 IC1.19
  Bottom 0.254: v21.59,11.33 24.41,11.33 24.51,11.43 v30.48,11.43
RXD0
  Top 0.254: IC2.34 26.04,25.4 25.14,24.51 25.14,14.98 26.06,14.06 26.06,13.56 28.32,11.3 28.7,11.3 28.82,11.18 IC1.21
SCL  (via drill 0.35)
  Top 0.152: 27.6,28 31.17,28 31.57,28.39 31.57,28.64
  Top 0.254: R10.1 32.13,34.84 v32.13,33.4 | IC2.36 27.6,28 | IC3.23 31.75,28.46 31.57,28.64 31.14,29.07 v31.14,29.34
  Bottom 0.254: v31.14,29.34 32.13,30.33 v32.13,33.4
SDA  (via drill 0.35)
  Top 0.254: IC3.24 32.3,27.94 31.77,27.94 v31.13,27.3 | R11.1 28.88,33.62 28.88,29.64 28.83,29.59 | IC2.37 27.67,29.34 28.57,29.34 28.83,29.59 | 28.83,29.59 28.83,28.84 v29.07,28.6
  Bottom 0.254: v29.07,28.6 29.83,28.6 v31.13,27.3
TXD0  (via drill 0.51)
  Top 0.254: IC2.35 26.04,26.67 24.64,25.27 24.64,14.8 25.63,13.81 25.63,12.65 v25.78,12.5 | v28.57,12.19 29.32,11.44 IC1.20
  Bottom 0.254: v28.57,12.19 28.27,12.5 v25.78,12.5
VBAT  (via drill 0.35, 0.51)
  Top 0.254: 15.24,15.24 v15.31,15.24
  Top 0.406: S2.3 5.04,25.44 5.88,24.6 5.88,23.37 | 5.88,23.37 R3.2 | 5.88,23.37 v7.62,23.37 | v14.61,22.86 14.61,20.32 v15.88,19.05 15.88,15.88 15.24,15.24 | v30.1,18.92 30.97,19.8 33.68,19.8 Q1.3 | v15.24,6.35 C7.1 14.31,3.9 13.84,3.43 13.84,2.29 13.18,1.62 U3.3
  Bottom 0.254: v15.88,19.05 16,18.92 | v15.31,15.24 15.24,15.17
  Bottom 0.406: v14.61,22.86 14.1,23.37 v7.62,23.37 | v30.1,18.92 16,18.92 | 15.24,15.17 v15.24,6.35
VBUS  (via drill 0.35, 0.51)
  Top 0.254: 31.46,16.52 R1.2 31.37,16.13 31.37,15.62 | v30.75,20.69 30.66,20.77 | R6.2 27.85,4.83 | v26.29,6.48 26.29,6.39
  Top 0.406: Q1.1 32.23,17.3 | 32.23,17.3 31.46,16.52 | 32.23,17.3 31.75,17.78 v31.75,18.41 | 30.66,20.77 D1.A | v9.27,4.45 8.64,4.45 7.35,5.73 LED1.A C14.1 | v11.08,4.54 11.68,4.54 U3.4 12.66,4.22 v13.52,5.08 | v19.7,6.73 20.65,7.69 D2.2 21,6.84 20.04,5.88 J1.1 | 27.85,4.83 26.29,6.39 | v32.03,12.28 32.38,12.64 32.38,14.61 31.37,15.62
  Bottom 0.254: v31.75,18.41 31.72,18.44 31.72,18.67 | 10.98,4.45 v11.08,4.54
  Bottom 0.406: 31.72,18.67 30.75,19.64 v30.75,20.69 | v9.27,4.45 10.98,4.45 | 24.43,5.61 23.82,5.61 22.96,6.48 22.71,6.73 v19.7,6.73 18.04,5.08 v13.52,5.08 | v26.29,6.48 25.3,6.48 24.43,5.61 | 24.43,5.61 31.01,5.61 32.51,7.11 32.51,11.8 v32.03,12.28

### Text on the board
tPlace: X | Y | Z
bPlace: GliderThrow_Meter - V1.0 - Alain Désandré - Avril 2020 | see https://gliderthrow-meter.readthedocs.io/en/latest/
